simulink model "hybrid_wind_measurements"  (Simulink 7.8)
settings: Solver=FixedStepDiscrete  SolverMode=SingleTasking  StartTime=0.0  StopTime=inf  FixedStep=Ts  RelTol=1e-3
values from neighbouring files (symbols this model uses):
  amp_gain_factor = 0.73316    [hybrid_wind.m]    (also in measurements.m = 0.73312)
  Ampl_chirp = maxoutputvoltage/4    (= 1.25)    [measurements.m]
  Ampl_chirp_F = maxLSvolts*Bl/Re    [measurements.m]
  Ampl_chirp_U = maxoutputvoltage *amp_gain_factor*Bl/Re/(2*pi*fstop)*Sd/Mms    [measurements.m]
  HLL_d = c2d(HLL_c,Ts)    [hybrid_wind.m]    (also in measurements.m)
  maxoutputvoltage = 5    [hybrid_wind.m]    (also in measurements.m)
  micoffset_V = mean(voltsin_calib)    [hybrid_wind.m]    (also in measurements.m)
  micpreampsensitivity = -0.0025726    [hybrid_wind.m]    (also in measurements.m)
  sweep_time = runtime    (= 20)    [measurements.m]
  Ts = 25e-6    (= 2.5e-05)    [hybrid_wind.m]    (also in measurements.m)
undefined symbols (not defined in the file or in its folder): Bl, cell2mat, Mms, Re, Sd
libraries: dspsrcs4 x3, simulink x1

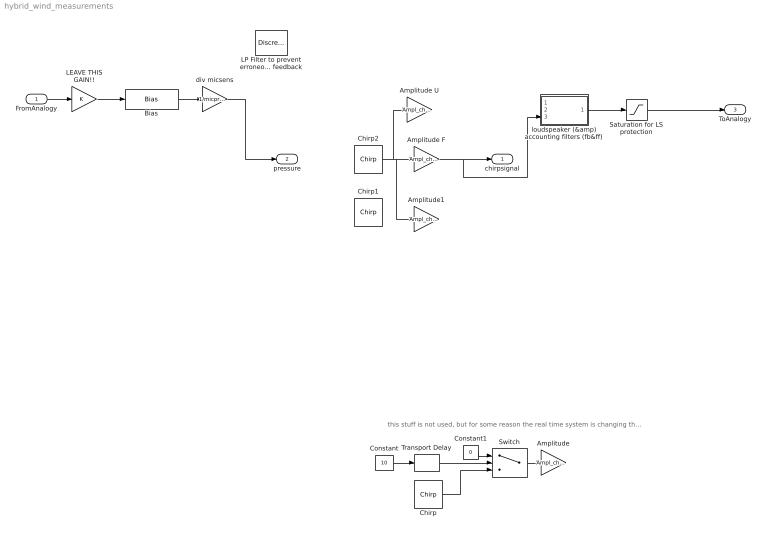
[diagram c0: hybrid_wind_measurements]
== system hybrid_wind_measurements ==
  note: this stuff is not used, but for some reason the real time system is changing the execution timing when the simulink patch is not complex enough!!
  FromAnalogy : Inport
  Amplitude : Gain  Gain=Ampl_chirp
  Amplitude F : Gain  Gain=Ampl_chirp_F
  Amplitude U : Gain  Gain=Ampl_chirp_U
  Amplitude1 : Gain  Gain=Ampl_chirp
  Bias : Bias  Bias=-micoffset_V
  Chirp : dspsrcs4/Chirp  sweep=Linear  mode=Unidirectional  f0=fstart  f1=fstop  t1=sweep_time  Tsweep=sweep_time  phase=pi/2  Ts=Ts  spf=1  datatype=Single
  Chirp1 : dspsrcs4/Chirp  sweep=Linear  mode=Unidirectional  f0=fstart  f1=fstop  t1=sweep_time  Tsweep=sweep_time  phase=pi/2  Ts=Ts  spf=1  datatype=Double
  Chirp2 : dspsrcs4/Chirp  sweep=Logarithmic  mode=Unidirectional  f0=fstart  f1=fstop  t1=sweep_time  Tsweep=sweep_time  phase=pi/2  Ts=Ts  spf=1  datatype=Double
  Constant : Constant  Value=10
  Constant1 : Constant  Value=0
  LEAVE THIS GAIN!! : Gain
  LP Filter to prevent erroneous high freq feedback : DiscreteFilter  Numerator=HdLP.ScaleValues(1)*HdLP.sosMatrix(1:end/2)  Denominator=HdLP.ScaleValues(2)*HdLP.sosMatrix(1+end/2:end)  SampleTime=Ts
  Saturation for LS protection : Saturate  UpperLimit=maxoutputvoltage  LowerLimit=-maxoutputvoltage
  Switch : Switch  Threshold=1
  Transport Delay : TransportDelay  DelayTime=sweep_time  BufferSize=8
  div micsens : Gain  Gain=1/micpreampsensitivity
  loudspeaker (&amp) accounting filters (fb&ff) : Subsystem
  chirpsignal : Outport
  pressure : Outport  Port=2
  ToAnalogy : Outport  Port=3
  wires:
  Chirp2/1 -> Amplitude F/1, Amplitude1/1, Amplitude U/1
  Constant/1 -> Transport Delay/1
  Transport Delay/1 -> Switch/2
  Constant1/1 -> Switch/1
  Switch/1 -> Amplitude/1
  Chirp/1 -> Switch/3
  Amplitude/1 -> ?
  Saturation for LS protection/1 -> ToAnalogy/1
  loudspeaker (&amp) accounting filters (fb&ff)/1(V_amp_in) -> Saturation for LS protection/1
  Amplitude F/1 -> loudspeaker (&amp) accounting filters (fb&ff)/3(FLS), chirpsignal/1
  div micsens/1 -> pressure/1
  Bias/1 -> div micsens/1
  FromAnalogy/1 -> LEAVE THIS GAIN!!/1
  LEAVE THIS GAIN!!/1 -> Bias/1

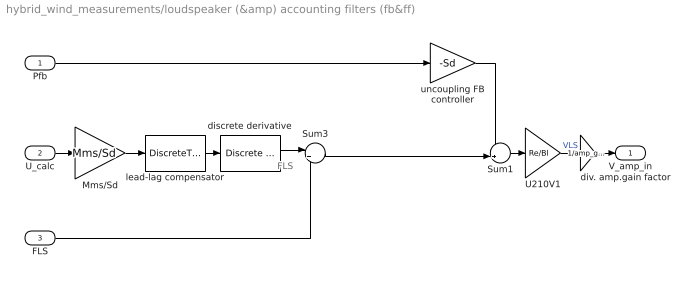
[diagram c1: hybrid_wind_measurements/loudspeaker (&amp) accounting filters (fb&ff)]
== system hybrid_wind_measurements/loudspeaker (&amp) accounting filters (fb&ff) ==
  note: FLS
  Pfb : Inport
  U_calc : Inport  Port=2
  FLS : Inport  Port=3
  Mms/Sd : Gain  Gain=Mms/Sd
  Sum1 : Sum  Inputs=-+|
  Sum3 : Sum  Inputs=|++
  U210V1 : Gain  Gain=Re/Bl
  discrete derivative : simulink/Discrete/Discrete Derivative  gainval=1.0  ICPrevScaledInput=0.0  InputProcessing=Inherited  OutMin=[]  OutMax=[]  OutDataType=fixdt(1, 16)  OutScaling=2^-10  DoSatur=off
  div. amp.gain factor : Gain  Gain=1/amp_gain_factor
  lead-lag compensator : DiscreteTransferFcn  Numerator=cell2mat(HLL_d.num)  Denominator=cell2mat(HLL_d.den)  SampleTime=Ts
  uncoupling FB controller : Gain  Gain=-Sd
  V_amp_in : Outport
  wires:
  Sum1/1 -> U210V1/1
  U210V1/1 -> div. amp.gain factor/1  "VLS"
  U_calc/1 -> Mms/Sd/1
  Pfb/1 -> uncoupling FB controller/1
  Mms/Sd/1 -> lead-lag compensator/1
  lead-lag compensator/1 -> discrete derivative/1
  div. amp.gain factor/1 -> V_amp_in/1
  Sum3/1 -> Sum1/2
  FLS/1 -> Sum3/2
  discrete derivative/1 -> Sum3/1
  uncoupling FB controller/1 -> Sum1/1
